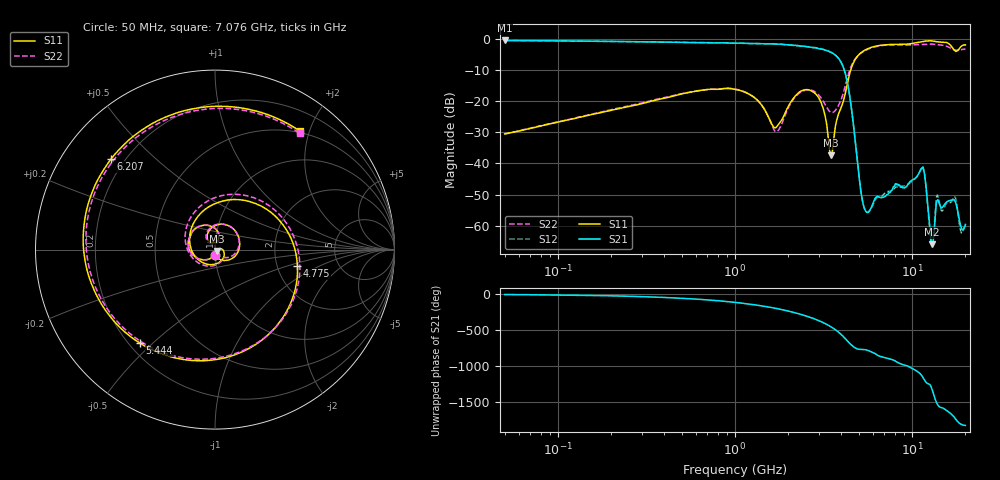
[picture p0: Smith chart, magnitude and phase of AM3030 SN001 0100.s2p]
# Hz S DB R 50
!freq MagS11 AngS11 MagS21 AngS21 MagS12 AngS12 MagS22 AngS22
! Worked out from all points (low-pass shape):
!   1601 points, 50 MHz to 20.05 GHz, reference 50 ohm
!   highest |S21| = -0.42 dB at 50 MHz (marker M1); lowest = -66.0 dB at 12.98 GHz (marker M2)
!   |S21| within 3 dB of the highest: start of sweep to 3.197 GHz
!   lowest |S11| = -37.4 dB at 3.499 GHz (marker M3), VSWR 1.03, Z = 51.1 - j0.762 ohm
!   |S11| at or under -10 dB: start of sweep to 4.507 GHz
!   |S22| runs from -30.5 to -1.6 dB; largest |S21 - S12| = 0.015
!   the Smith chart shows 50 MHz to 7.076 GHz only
!   S11 on the Smith chart (normalised r, x): 50 MHz: 1.00, -0.06; 4.775 GHz: 2.60, -0.60; 5.444 GHz: 0.24, -0.46; 6.207 GHz: 0.15, +0.37; 7.076 GHz: 0.48, +1.85
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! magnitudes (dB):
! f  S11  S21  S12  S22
! 50 MHz  -30.5  -0.4  -0.4  -30.5
! 135.9 MHz  -25.0  -0.6  -0.6  -24.9
! 369.6 MHz  -19.4  -0.9  -0.9  -19.2
! 1.005 GHz  -16.2  -1.3  -1.3  -16.1
! 1.351 GHz  -19.9  -1.4  -1.5  -19.8
! 1.717 GHz  -28.3  -1.6  -1.6  -29.7
! 2.191 GHz  -18.3  -2.0  -2.1  -18.6
! 2.722 GHz  -16.7  -2.7  -2.6  -16.5
! 3.127 GHz  -21.7  -3.3  -3.2  -19.6
! 3.499 GHz  -37.4  -4.3  -4.3  -23.6
! 4.188 GHz  -17.9  -10.7  -10.7  -15.4
! 4.775 GHz  -6.6  -32.3  -32.3  -6.4
! 5.444 GHz  -3.5  -55.0  -55.0  -3.7
! 6.207 GHz  -2.3  -51.1  -51.7  -2.5
! 7.076 GHz  -1.8  -50.6  -49.4  -1.9
! 7.402 GHz  -1.7  -49.5  -49.1  -1.9
! 11.47 GHz  -0.8  -41.3  -40.9  -1.7
! 12.98 GHz  -0.6  -66.0  -66.6  -1.6
! 13.99 GHz  -0.9  -51.7  -50.3  -1.8
! 17.39 GHz  -3.6  -51.8  -50.6  -3.4
! 18.95 GHz  -2.4  -60.4  -62.1  -3.4
! 20.05 GHz  -1.9  -59.6  -59.7  -3.2
